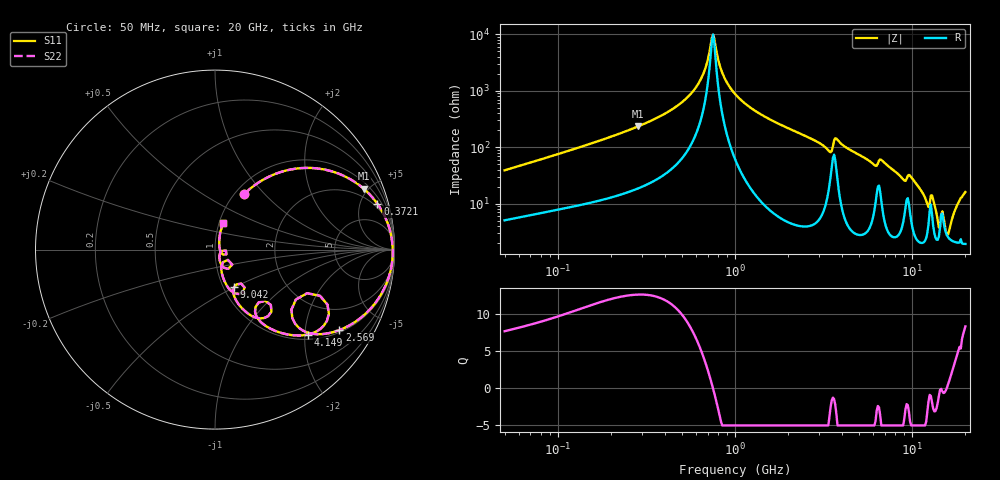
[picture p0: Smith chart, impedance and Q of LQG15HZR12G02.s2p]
!Murata Part Number: LQG15HZR12G02
!These Parameters are Measured in Series Mode Connection
!  o--[Z]--o
!Port1  Port2
!  o-------o
!Freq. Start=50[MHz] Stop=20[GHz], 401[Steps]
# Hz S RI R 50
!Freq.(Hz) S11(Real) S11(Imag) S21(Real) S21(Imag) S12(Real) S12(Imag) S22(Real) S22(Imag)
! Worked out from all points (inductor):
!   401 points, 50 MHz to 20 GHz, reference 50 ohm
!   read as one part in series: L = 120 nH near 51.52 MHz
!   highest Q = 12.5 at 284.2 MHz (marker M1), where L = 131 nH
!   self-resonance near 741.1 MHz
!   S11 on the Smith chart (normalised r, x): 50 MHz: 1.10, +0.77; 372.1 MHz: 1.57, +6.90; 2.569 GHz: 1.08, -3.04; 4.149 GHz: 1.11, -2.07; 9.042 GHz: 1.12, -0.50; 20 GHz: 1.04, +0.32
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5e7  0.1617 0.3084  0.8383 -0.3084  0.8383 -0.3084  0.1617 0.3084
1.364002e8  0.513 0.4553  0.487 -0.4553  0.487 -0.4553  0.513 0.4553
2.841629e8  0.8278 0.3399  0.1722 -0.3399  0.1722 -0.3399  0.8278 0.3399
3.721004e8  0.9052 0.2547  0.0948 -0.2547  0.0948 -0.2547  0.9052 0.2547
6.009314e8  0.9803 0.0834  0.0197 -0.0834  0.0197 -0.0834  0.9803 0.0834
6.673612e8  0.9868 0.0443  0.0132 -0.0443  0.0132 -0.0443  0.9868 0.0443
7.523192e8  0.9901 -0.00073  0.00986 0.00073  0.00986 0.00073  0.9901 -0.00073
8.608917e8  0.9885 -0.052  0.0115 0.052  0.0115 0.052  0.9885 -0.052
1e9  0.9799 -0.1097  0.0201 0.1097  0.0201 0.1097  0.9799 -0.1097
2.569357e9  0.6935 -0.4482  0.3065 0.4482  0.3065 0.4482  0.6935 -0.4482
2.728004e9  0.6548 -0.4608  0.3452 0.4608  0.3452 0.4608  0.6548 -0.4608
3.572216e9  0.5134 -0.243  0.4866 0.243  0.4866 0.243  0.5134 -0.243
4.149438e9  0.5173 -0.4733  0.4827 0.4733  0.4827 0.4733  0.5173 -0.4733
7.442007e9  0.1816 -0.3545  0.8184 0.3545  0.8184 0.3545  0.1816 -0.3545
9.041845e9  0.1067 -0.2094  0.8933 0.2094  0.8933 0.2094  0.1067 -0.2094
9.892087e9  0.114 -0.2449  0.886 0.2449  0.886 0.2449  0.114 -0.2449
1.220001e10  0.0373 -0.0873  0.9627 0.0873  0.9627 0.0873  0.0373 -0.0873
1.314879e10  0.0501 -0.1012  0.9499 0.1012  0.9499 0.1012  0.0501 -0.1012
1.396067e10  0.0242 -0.0429  0.9758 0.0429  0.9758 0.0429  0.0242 -0.0429
1.504638e10  0.0469 -0.0286  0.9531 0.0286  0.9531 0.0286  0.0469 -0.0286
1.573793e10  0.0268 0.0021  0.9732 -0.0021  0.9732 -0.0021  0.0268 0.0021
2e10  0.0424 0.1501  0.9576 -0.1501  0.9576 -0.1501  0.0424 0.1501
